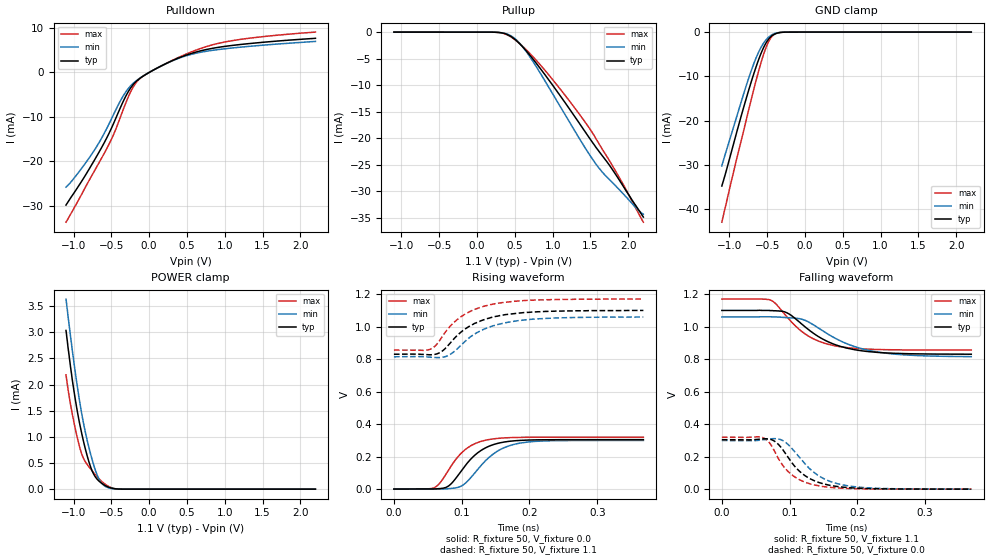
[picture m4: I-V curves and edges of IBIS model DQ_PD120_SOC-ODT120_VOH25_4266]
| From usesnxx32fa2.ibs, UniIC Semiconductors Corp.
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| DQ_PD120_SOC-ODT120_VOH25_4266
| (120 Ohm Pulldown, 120 Ohm System ODT Setting, VOH=VDDQ/2.5, 3200-4266Mbps)
[Model]   DQ_PD120_SOC-ODT120_VOH25_4266
Model_type   I/O
Vinl = 160.000mV
Vinh = 280.000mV
Vmeas = 220.000mV
Vref = 0.0mV
Cref = 0.0pF
Rref = 120.000Ohm
|   typ   min   max
|C_comp   0.834pF   0.784pF   0.884pF
C_comp_pullup   0.4170pF   0.3920pF   0.4420pF
C_comp_pulldown   0.4170pF   0.3920pF   0.4420pF
| Note: C_comp changes when the ODT circuit is enabled.
[Model Spec]
| Input threshold voltage corners
Vinl   0.1600V   0.1520V   0.1740V
Vinh   0.2800V   0.2720V   0.2940V
| Measurement voltage corners
Vmeas   0.2200V   0.2120V   0.2340V
| Timing spec test load voltage corners
Vref   0.0000V   0.0000V   0.0000V
| Dynamic Overshoot Parameters from LPDDR4 Specification
D_overshoot_ampl_h   0.30   NA   NA
D_overshoot_ampl_l   0.30   NA   NA
D_overshoot_area_h   0.1n   NA   NA
D_overshoot_area_l   0.1n   NA   NA
[Voltage Range]   1.1000V   1.0600V   1.1700V
[Pullup Reference]   1.1000V   1.0600V   1.1700V
| Junction Temperature (Ambient temp is 35C typ 95C min -40C max)
[Temperature Range]   50.0   110.0   -40.0
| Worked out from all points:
|   slope of the pulldown table from 0 to 0.165 V, typ, clamps not added: 109 ohm
|   slope of the pullup table from 0 to 0.165 V, typ, clamps not added: 26.6 kohm
|   GND clamp passes 1 mA (typ) near -0.45 V on its own axis
|   POWER clamp passes 1 mA (typ) near -0.88 V on its own axis
|   rising waveform, R_fixture 50, V_fixture 0.0: 20-80 % time 40.3ps typ, 44ps min, 36.8ps max; typ from 0.001 V to 0.305 V
|   falling waveform, R_fixture 50, V_fixture 1.1: 20-80 % time 61.1ps typ, 71.1ps min, 51.7ps max; typ from 1.1 V to 0.831 V
|   rising waveform, R_fixture 50, V_fixture 1.1: 20-80 % time 55.1ps typ, 57.5ps min, 51.5ps max; typ from 0.83 V to 1.1 V
|   falling waveform, R_fixture 50, V_fixture 0.0: 20-80 % time 41.8ps typ, 47ps min, 37.1ps max; typ from 0.305 V to 0.001 V
[Pulldown]
|   Voltage   I(typ)   I(min)   I(max)
-1.1V     -29.87mA   -25.83mA   -33.73mA
-935mV    -25.62mA   -22.54mA   -28.77mA
-707.3mV  -19.27mA   -17.05mA   -21.68mA
-486.2mV  -12.09mA   -10.02mA   -14.59mA
-380.6mV  -7.948mA   -6.414mA   -10.08mA
-304.7mV  -5.221mA   -4.289mA   -6.699mA
-202.4mV  -2.585mA   -2.33mA    -3.06mA
-100.1mV  -1.078mA   -1.043mA   -1.096mA
398.2mV   3.296mA    3.212mA    3.438mA
830.5mV   5.391mA    4.945mA    6.165mA
1.306V    6.452mA    5.831mA    7.652mA
2.2V      7.669mA    6.972mA    9.07mA
[GND Clamp]
|   Voltage   I(typ)   I(min)   I(max)
-1.1V     -34.75mA   -30.21mA   -42.92mA
-1.037V   -31.05mA   -26.58mA   -38.3mA
-944.9mV  -25.23mA   -21.44mA   -31.56mA
-789.8mV  -15.73mA   -12.78mA   -20.73mA
-664.4mV  -8.74mA    -6.576mA   -12.08mA
-588.5mV  -5.115mA   -3.68mA    -7.305mA
-522.5mV  -2.666mA   -1.903mA   -3.813mA
-469.7mV  -1.356mA   -986.1uA   -1.787mA
-413.6mV  -565.1uA   -416.4uA   -620.7uA
-347.6mV  -154.3uA   -117.4uA   -135.5uA
-251.9mV  -13.38uA   -11.89uA   -7.924uA
2.2V      0A         0A         0A
[Pullup]
|   Voltage   I(typ)   I(min)   I(max)
-1.1V     2.737uA    4.954uA    907.4nA
266.2mV   -46.06uA   -45.34uA   -47.87uA
391.6mV   -403.2uA   -334.2uA   -479.9uA
497.2mV   -1.328mA   -1.186mA   -1.397mA
606.1mV   -2.828mA   -2.823mA   -2.719mA
748mV     -5.234mA   -5.722mA   -4.774mA
1.108V    -12.17mA   -14.22mA   -10.89mA
1.441V    -19.03mA   -22.09mA   -17.2mA
1.655V    -23.3mA    -26.38mA   -22.06mA
1.933V    -29.06mA   -30.5mA    -28.72mA
2.121V    -33.18mA   -33.4mA    -33.8mA
2.2V      -34.89mA   -34.36mA   -35.86mA
[POWER Clamp]
|   Voltage   I(typ)   I(min)   I(max)
-1.1V     3.033mA    3.633mA    2.184mA
-1.041V   2.345mA    2.929mA    1.625mA
-968mV    1.637mA    2.139mA    1.094mA
-905.3mV  1.155mA    1.553mA    732.3uA
-845.9mV  779.9uA    1.103mA    527.4uA
-773.3mV  420.7uA    665.2uA    384.1uA
-707.3mV  225.5uA    345.4uA    267.6uA
-651.2mV  138.6uA    162.4uA    181.2uA
-591.8mV  77.92uA    64.83uA    105.5uA
-499.4mV  21.32uA    13.13uA    27.43uA
-400.4mV  2.57uA     1.7uA      2.311uA
2.2V      0A         0A         0A
[Ramp]
|   typ   min   max
| 20% - 80%
dV/dt_r   182.47m/40.32p   179.53m/44.00p   191.77m/36.76p
dV/dt_f   161.58m/61.12p   146.48m/71.15p   188.38m/51.71p
| 25% - 75%
|dV/dt_r   152.06m/32.10p   149.61m/35.06p   159.81m/29.23p
|dV/dt_f   134.65m/48.61p   122.06m/56.66p   156.98m/41.00p
R_load = 50
[Rising Waveform]
R_fixture = 50
V_fixture = 0.0
|   Time   V(typ)   V(min)   V(max)
0s        649.5uV    533.1uV    475.6uV
58ps      810.3uV    43.63uV    6.641mV
67ps      3.137mV    61.69uV    34.11mV
77ps      11.22mV    1.86mV     93.61mV
103ps     133.1mV    28.37mV    235.8mV
118ps     203.9mV    93.33mV    277mV
136ps     256.1mV    178.6mV    302mV
162ps     289.6mV    254.2mV    315.3mV
194ps     301.6mV    288.5mV    319.2mV
368ps     304.8mV    299.7mV    320.1mV
[Falling Waveform]
R_fixture   = 50
V_fixture   = 1.1
V_fixture_min = 1.06
V_fixture_max = 1.17
|   Time   V(typ)   V(min)   V(max)
0s        1.1V       1.06V      1.17V
73ps      1.099V     1.061V     1.162V
81ps      1.097V     1.06V      1.135V
96ps      1.086V     1.056V     1.061V
120ps     1.009V     1.043V     963.9mV
142ps     940.4mV    993.1mV    912.3mV
164ps     894.5mV    936.3mV    884.7mV
200ps     855.5mV    872.2mV    865.4mV
239ps     839.4mV    838.6mV    858.8mV
368ps     830.7mV    815.9mV    856mV
[Rising Waveform]
R_fixture   = 50
V_fixture   = 1.1
V_fixture_min = 1.06
V_fixture_max = 1.17
|   Time   V(typ)   V(min)   V(max)
0s        830.4mV    814.6mV    855.9mV
55ps      827.1mV    811.8mV    863.9mV
62ps      830.9mV    809.8mV    886mV
71ps      848.9mV    811.2mV    937.1mV
82ps      894.1mV    826.8mV    998.2mV
94ps      948.6mV    865.8mV    1.046V
118ps     1.018V     952.1mV    1.104V
146ps     1.059V     1.005V     1.139V
214ps     1.092V     1.049V     1.165V
368ps     1.1V       1.06V      1.17V
[Falling Waveform]
R_fixture = 50
V_fixture = 0.0
|   Time   V(typ)   V(min)   V(max)
0s        304.9mV    299.8mV    320.2mV
61ps      310.1mV    304mV      316.5mV
71ps      307.7mV    309.6mV    281.8mV
87ps      259.2mV    305mV      164.2mV
99ps      188.4mV    270.3mV    104.1mV
113ps     116.8mV    202.9mV    62.03mV
141ps     44.75mV    87.97mV    22.53mV
167ps     18.77mV    38.26mV    9.045mV
201ps     6.396mV    13.29mV    2.96mV
368ps     748.6uV    711.3uV    514.3uV
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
